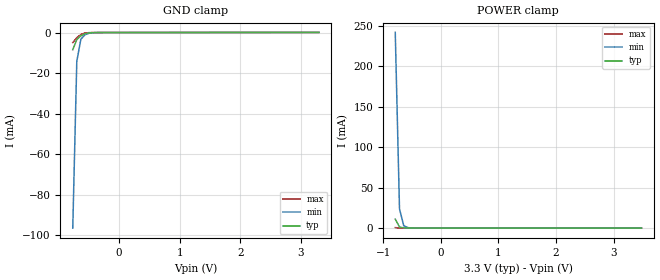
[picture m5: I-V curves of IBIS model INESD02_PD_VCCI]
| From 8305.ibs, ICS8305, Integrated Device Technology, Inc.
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[Model] INESD02_PD_VCCI
Model_type   Input
Polarity   Non-Inverting
Vinl = 0.8V
Vinh = 2.0V
|   typ   min   max
C_comp   2pF   1.5pF   2.5pF
|   typ   min   max
[Voltage range]   3.3V   3.135V   3.465V
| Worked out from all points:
|   GND clamp passes 1 mA (typ) near -0.59 V on its own axis
|   POWER clamp passes 1 mA (typ) near -0.70 V on its own axis
[GND_clamp]
|Voltage   I (typ)   I (min)   I (max)
|Note, modeling breaks down at 250mA and above.  This is well beyond the functional   |
|operating range of the device.  Should this scenario occur, catastrophic failure and   |
|possible damage to the device and/or board is of higher concern than the I-V curve   |
|behavior.  The IBIS checker will flag currents in excess of 10A with warnings.  Lines   |
|with currents in excess of 0.35 A have been commented out.  The points still remain|
|available to the user if the user desires to use them.   |
|-3.30000e+00   -1.45240e+01   -1.25449e+01   -1.78533e+01
|-3.23333e+00   -1.41303e+01   -1.22167e+01   -1.73507e+01
|-3.16667e+00   -1.37365e+01   -1.18884e+01   -1.68482e+01
|-3.10000e+00   -1.33428e+01   -1.15602e+01   -1.63456e+01
|-3.03333e+00   -1.29491e+01   -1.12320e+01   -1.58431e+01
|-2.96667e+00   -1.25554e+01   -1.09037e+01   -1.53405e+01
|-2.90000e+00   -1.21617e+01   -1.05755e+01   -1.48380e+01
|-2.83333e+00   -1.17680e+01   -1.02473e+01   -1.43354e+01
|-2.76667e+00   -1.13743e+01   -9.91905e+00   -1.38328e+01
|-2.70000e+00   -1.09806e+01   -9.59084e+00   -1.33303e+01
|-2.63333e+00   -1.05869e+01   -9.26262e+00   -1.28277e+01
|-2.56667e+00   -1.01932e+01   -8.93441e+00   -1.23251e+01
|-2.50000e+00   -9.79944e+00   -8.60620e+00   -1.18225e+01
|-2.43333e+00   -9.40572e+00   -8.27799e+00   -1.13199e+01
|-2.36667e+00   -9.01201e+00   -7.94979e+00   -1.08173e+01
|-2.30000e+00   -8.61829e+00   -7.62159e+00   -1.03147e+01
|-2.23333e+00   -8.22457e+00   -7.29339e+00   -9.81212e+00
|-2.16667e+00   -7.83084e+00   -6.96520e+00   -9.30950e+00
|-2.10000e+00   -7.43712e+00   -6.63701e+00   -8.80687e+00
|-2.03333e+00   -7.04340e+00   -6.30883e+00   -8.30423e+00
|-1.96667e+00   -6.64967e+00   -5.98065e+00   -7.80159e+00
|-1.90000e+00   -6.25595e+00   -5.65249e+00   -7.29894e+00
|-1.83333e+00   -5.86224e+00   -5.32433e+00   -6.79628e+00
|-1.76667e+00   -5.46852e+00   -4.99619e+00   -6.29362e+00
|-1.70000e+00   -5.07482e+00   -4.66807e+00   -5.79096e+00
|-1.63333e+00   -4.68113e+00   -4.33997e+00   -5.28829e+00
|-1.56667e+00   -4.28745e+00   -4.01189e+00   -4.78563e+00
|-1.50000e+00   -3.89380e+00   -3.68384e+00   -4.28297e+00
|-1.43333e+00   -3.50017e+00   -3.35583e+00   -3.78032e+00
|-1.36667e+00   -3.10657e+00   -3.02786e+00   -3.27769e+00
|-1.30000e+00   -2.71302e+00   -2.69994e+00   -2.77509e+00
|-1.23333e+00   -2.31953e+00   -2.37209e+00   -2.27252e+00
|-1.16667e+00   -1.92610e+00   -2.04430e+00   -1.77000e+00
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-766.7mV  -8.501mA   -96.61mA   -4.97mA
-700mV    -3.491mA   -14.25mA   -2.553mA
-633.3mV  -1.625mA   -3.336mA   -976.6uA
-566.7mV  -614uA     -1.128mA   -263.9uA
-500mV    -180.1uA   -382.8uA   -57.92uA
-300mV    -6.78uA    -12.51uA   -4.58uA
3.3V      64.29uA    80.43uA    49.82uA
[Power_clamp]
|Voltage   I (typ)   I (min)   I (max)
|Note, modeling breaks down at 250mA and above.  This is well beyond the functional   |
|operating range of the device.  Should this scenario occur, catastrophic failure and   |
|possible damage to the device and/or board is of higher concern than the I-V curve   |
|behavior.  The IBIS checker will flag currents in excess of 10A with warnings.  Lines   |
|with currents in excess of 0.35 A have been commented out.  The points still remain|
|available to the user if the user desires to use them.   |
|-3.30000e+00   2.53699e+01   2.18883e+01   3.12330e+01
|-3.22626e+00   2.46049e+01   2.12511e+01   3.02556e+01
|-3.15253e+00   2.38398e+01   2.06136e+01   2.92783e+01
|-3.07879e+00   2.30748e+01   1.99762e+01   2.83010e+01
|-3.00505e+00   2.23097e+01   1.93388e+01   2.73237e+01
|-2.93131e+00   2.15447e+01   1.87014e+01   2.63463e+01
|-2.85758e+00   2.07797e+01   1.80640e+01   2.53690e+01
|-2.78384e+00   2.00147e+01   1.74267e+01   2.43917e+01
|-2.71010e+00   1.92497e+01   1.67894e+01   2.34144e+01
|-2.63636e+00   1.84847e+01   1.61521e+01   2.24370e+01
|-2.56263e+00   1.77197e+01   1.55148e+01   2.14597e+01
|-2.48889e+00   1.69548e+01   1.48776e+01   2.04824e+01
|-2.41515e+00   1.61899e+01   1.42404e+01   1.95051e+01
|-2.34141e+00   1.54250e+01   1.36032e+01   1.85278e+01
|-2.26768e+00   1.46601e+01   1.29661e+01   1.75506e+01
|-2.19394e+00   1.38953e+01   1.23290e+01   1.65733e+01
|-2.12020e+00   1.31305e+01   1.16920e+01   1.55961e+01
|-2.04646e+00   1.23657e+01   1.10550e+01   1.46189e+01
|-1.97273e+00   1.16010e+01   1.04180e+01   1.36418e+01
|-1.89899e+00   1.08364e+01   9.78110e+00   1.26647e+01
|-1.82525e+00   1.00718e+01   9.14426e+00   1.16876e+01
|-1.75152e+00   9.30727e+00   8.50748e+00   1.07106e+01
|-1.67778e+00   8.54283e+00   7.87078e+00   9.73376e+00
|-1.60404e+00   7.77848e+00   7.23416e+00   8.75696e+00
|-1.53030e+00   7.01422e+00   6.59763e+00   7.78028e+00
|-1.45657e+00   6.25009e+00   5.96120e+00   6.80373e+00
|-1.38283e+00   5.48609e+00   5.32488e+00   5.82734e+00
|-1.30909e+00   4.72224e+00   4.68868e+00   4.85114e+00
|-1.23535e+00   3.95857e+00   4.05263e+00   3.87517e+00
|-1.16162e+00   3.19509e+00   3.41673e+00   2.89946e+00
|-1.08788e+00   2.43185e+00   2.78101e+00   1.92408e+00
|-1.01414e+00   1.66887e+00   2.14548e+00   9.49091e-01
|-9.40404e-01   9.06212e-01   1.51018e+00   9.06225e-02
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-792.9mV  11.17mA    241.8mA    591.9uA
-719.2mV  1.314mA    23.75mA    171.6uA
-645.5mV  320.8uA    2.909mA    80.7uA
-571.7mV  126.1uA    559.8uA    63.41uA
-424.2mV  73.96uA    106.3uA    58.73uA
3.484V    -3.602uA   -25.3uA    -284.4nA
